| Teraspeed Modeling Services.
| http://www.teraspeedlabs.com
[IBIS Ver]   4.0
[Comment Char] |_char
[File Name]   lpc54114j256bd64.ibs
[File Rev]   3.0
[Source]  Measured and created by Teraspeed Labs
[Date]   10-25-2017
[Notes]   Quality Check of this IBIS model: Model Passes IBIS Check
   Model parses into ICX IS. Simulation done with Hyperlynx.
   1. MIN TYP MAX information is based on Temperature and Voltage
   characteristics only.
   2. Package data measured using Tektronix IConnect Software.
[Disclaimer]
| Use: Teraspeed Labs ("Teraspeed") has
| licensed IBIS models to specific integrated circuit
| suppliers ("IC Vendors") for use and distribution as
| follows: Each IC Vendor may use IBIS Models, and distribute
| them to IC Vendor's customers to use solely for developing
| printed circuit board designs. Users of this model may
| modify the IBIS model to suit its specific applications but
| rights to derivative works and such modifications shall belong
| to Teraspeed. No other distribution of these materials is
| permitted.
| DISCLAIMER OF WARRANTY: UNLESS OTHERWISE AGREED TO IN WRITING
| TERASPEED DISCLAIMS AND USER WAIVES ALL WARRANTIES, EXPRESS
| OR IMPLIED, INCLUDING WARRANTIES OF MERCHANTABILITY AND
| FITNESS FOR A PARTICULAR PURPOSE. IN NO EVENT SHALL
| TERASPEED BE LIABLE FOR ANY DIRECT OR INDIRECT DAMAGES,
| WHETHER IN CONTRACT OR TORT, INCLUDING, WITHOUT LIMITATION,
| LOST PROFITS, BUSINESS INTERRUPTION, OR LOST INFORMATION
| ARISING OUT OF THE USE OF OR THE INABILITY TO USE THE MODEL,
| EVEN IF TERASPEED HAS BEEN ADVISED OF THE POSSIBILITY OF SUCH
| DAMAGES.
[Copyright]
| This file is the legal property of Teraspeed Labs Copyright(c) 2017.
| All other rights are reserved.
[Component] LPC54114J256BD64
[Manufacturer] NXP Semiconductors
| Data Sheet: Rev 1.2, 24 February 2016
[Package]
| variable   typ   min   max
| LQFP64/SOT314-2
R_pkg  6.050E-02  5.800E-02  6.500E-02
L_pkg  5.046E-09  4.850E-09  5.380E-09
C_pkg  2.675E-13  2.400E-13  3.000E-13
[Pin] signal_name  model_name  R_pin  L_pin C_pin
1   PIO0_23   pio0_23   6.500E-02   5.380E-09   3.000E-13
2   PIO0_24   pio0_24   6.300E-02   5.250E-09   2.900E-13
3   PIO0_25   pio0_25   6.200E-02   5.130E-09   2.800E-13
4   PIO0_26   pio0_26   6.000E-02   5.040E-09   2.700E-13
5   USB_DP   analog_io   5.900E-02   4.950E-09   2.600E-13
6   USB_DM   analog_io   5.900E-02   4.900E-09   2.500E-13
7   PIO1_16   pio1_16   5.800E-02   4.870E-09   2.500E-13
8   VDD   POWER   5.800E-02   4.850E-09   2.400E-13
9   VSS   GND   5.800E-02   4.850E-09   2.400E-13
10   PIO1_17   pio1_17   5.800E-02   4.870E-09   2.500E-13
11   PIO0_29/ADC0_0   pio0_29   5.900E-02   4.900E-09   2.500E-13
12   PIO0_30/ADC0_1   pio0_30   5.900E-02   4.950E-09   2.600E-13
13   PIO0_31/ADC0_2   pio0_31   6.000E-02   5.040E-09   2.700E-13
14   PIO1_0/ADC0_3   pio1_0   6.200E-02   5.130E-09   2.800E-13
15   PIO1_1/ADC0_4   pio1_1   6.300E-02   5.250E-09   2.900E-13
16   PIO1_2/ADC0_5   pio1_2   6.500E-02   5.380E-09   3.000E-13
17   PIO1_3/ADC0_6   pio1_3   6.500E-02   5.380E-09   3.000E-13
18   PIO1_4/ADC0_7   pio1_4   6.300E-02   5.250E-09   2.900E-13
19   PIO1_5/ADC0_8   pio1_5   6.200E-02   5.130E-09   2.800E-13
20   VSSA   GND   6.000E-02   5.040E-09   2.700E-13
21   VREFN   GND   5.900E-02   4.950E-09   2.600E-13
22   VREFP   POWER   5.900E-02   4.900E-09   2.500E-13
23   VDDA   POWER   5.800E-02   4.870E-09   2.500E-13
24   VDD   POWER   5.800E-02   4.850E-09   2.400E-13
25   VSS   GND   5.800E-02   4.850E-09   2.400E-13
26   PIO1_6/ADC0_9   pio1_6   5.800E-02   4.870E-09   2.500E-13
27   PIO1_7/ADC0_10   pio1_7   5.900E-02   4.900E-09   2.500E-13
28   PIO1_8/ADC0_11   pio1_8   5.900E-02   4.950E-09   2.600E-13
29   PIO1_9   pio1_9   6.000E-02   5.040E-09   2.700E-13
30   PIO1_10   pio1_10   6.200E-02   5.130E-09   2.800E-13
31   PIO0_0   pio0_0   6.300E-02   5.250E-09   2.900E-13
32   PIO0_1   pio0_1   6.500E-02   5.380E-09   3.000E-13
33   RTCXIN   rtcxin   6.500E-02   5.380E-09   3.000E-13
34   VDD   POWER   6.300E-02   5.250E-09   2.900E-13
35   RTCXOUT   rtcxout   6.200E-02   5.130E-09   2.800E-13
36   PIO0_2   pio0_2   6.000E-02   5.040E-09   2.700E-13
37   PIO0_3   pio0_3   5.900E-02   4.950E-09   2.600E-13
38   PIO0_4   pio0_4   5.900E-02   4.900E-09   2.500E-13
39   PIO0_5   pio0_5   5.800E-02   4.870E-09   2.500E-13
40   PIO0_6   pio0_6   5.800E-02   4.850E-09   2.400E-13
41   PIO0_7   pio0_7   5.800E-02   4.850E-09   2.400E-13
42   PIO1_11   pio1_11   5.800E-02   4.870E-09   2.500E-13
43   PIO0_8   pio0_8   5.900E-02   4.900E-09   2.500E-13
44   PIO0_9   pio0_9   5.900E-02   4.950E-09   2.600E-13
45   PIO0_10   pio0_10   6.000E-02   5.040E-09   2.700E-13
46   PIO0_11   pio0_11   6.200E-02   5.130E-09   2.800E-13
47   PIO0_12   pio0_12   6.300E-02   5.250E-09   2.900E-13
48   PIO0_13   pio0_13   6.500E-02   5.380E-09   3.000E-13
49   PIO0_14/TCK   pio0_14   6.500E-02   5.380E-09   3.000E-13
50   PIO0_15/TDO   pio0_15   6.300E-02   5.250E-09   2.900E-13
51   PIO1_12   pio1_12   6.200E-02   5.130E-09   2.800E-13
52   SWCLK/PIO0_16   pio0_16   6.000E-02   5.040E-09   2.700E-13
53   SWDIO/PIO0_17   pio0_17   5.900E-02   4.950E-09   2.600E-13
54   PIO1_13   pio1_13   5.900E-02   4.900E-09   2.500E-13
55   VSS   GND   5.800E-02   4.870E-09   2.500E-13
56   VDD   POWER   5.800E-02   4.850E-09   2.400E-13
57   PIO1_14   pio1_14   5.800E-02   4.850E-09   2.400E-13
58   PIO0_18/*TRST   pio0_18   5.800E-02   4.870E-09   2.500E-13
59   PIO0_19/TDI   pio0_19   5.900E-02   4.900E-09   2.500E-13
60   PIO0_20/TMS   pio0_20   5.900E-02   4.950E-09   2.600E-13
61   PIO0_21   pio0_21   6.000E-02   5.040E-09   2.700E-13
62   PIO1_15   pio1_15   6.200E-02   5.130E-09   2.800E-13
63   PIO0_22   pio0_22   6.300E-02   5.250E-09   2.900E-13
64   *RESET   reset   6.500E-02   5.380E-09   3.000E-13
|**Open drain io pins
[Model Selector]   pio0_23
i2c_norm_hi_1.8v   i2c norm mode,hi drv,Open Drain io,1.8V
i2c_norm_hi_2.5v   i2c norm mode,hi drv,Open Drain io,2.5V
i2c_norm_hi_3.3v   i2c norm mode,hi drv,Open Drain io,3.3V
i2c_norm_lo_1.8v   i2c norm mode,lo drv,Open Drain io,1.8V
i2c_norm_lo_2.5v   i2c norm mode,lo drv,Open Drain io,2.5V
i2c_norm_lo_3.3v   i2c norm mode,lo drv,Open Drain io,3.3V
[Model Selector]   pio0_24
i2c_norm_hi_1.8v   i2c norm mode,hi drv,Open Drain io,1.8V
i2c_norm_hi_2.5v   i2c norm mode,hi drv,Open Drain io,2.5V
i2c_norm_hi_3.3v   i2c norm mode,hi drv,Open Drain io,3.3V
i2c_norm_lo_1.8v   i2c norm mode,lo drv,Open Drain io,1.8V
i2c_norm_lo_2.5v   i2c norm mode,lo drv,Open Drain io,2.5V
i2c_norm_lo_3.3v   i2c norm mode,lo drv,Open Drain io,3.3V
[Model Selector]   pio0_25
i2c_norm_hi_1.8v   i2c norm mode,hi drv,Open Drain io,1.8V
i2c_norm_hi_2.5v   i2c norm mode,hi drv,Open Drain io,2.5V
i2c_norm_hi_3.3v   i2c norm mode,hi drv,Open Drain io,3.3V
i2c_norm_lo_1.8v   i2c norm mode,lo drv,Open Drain io,1.8V
i2c_norm_lo_2.5v   i2c norm mode,lo drv,Open Drain io,2.5V
i2c_norm_lo_3.3v   i2c norm mode,lo drv,Open Drain io,3.3V
[Model Selector]   pio0_26
i2c_norm_hi_1.8v   i2c norm mode,hi drv,Open Drain io,1.8V
i2c_norm_hi_2.5v   i2c norm mode,hi drv,Open Drain io,2.5V
i2c_norm_hi_3.3v   i2c norm mode,hi drv,Open Drain io,3.3V
i2c_norm_lo_1.8v   i2c norm mode,lo drv,Open Drain io,1.8V
i2c_norm_lo_2.5v   i2c norm mode,lo drv,Open Drain io,2.5V
i2c_norm_lo_3.3v   i2c norm mode,lo drv,Open Drain io,3.3V
|**Standard io pins,5Vtol
[Model Selector]   pio0_0
pio_1.8v   GP io,1.8V
pio_2.5v   GP io,2.5V
pio_3.3v   GP io,3.3V
pio_1.8v_pd   GP io,pd,1.8V
pio_2.5v_pd   GP io,pd,2.5V
pio_3.3v_pd   GP io,pd,3.3V
pio_1.8v_pu   GP io,pu,1.8V | Pwrup Default
pio_2.5v_pu   GP io,pu,2.5V | Pwrup Default
pio_3.3v_pu   GP io,pu,3.3V | Pwrup Default
pio_fast_1.8v   GP io,fast slew,1.8V
pio_fast_2.5v   GP io,fast slew,2.5V
pio_fast_3.3v   GP io,fast slew,3.3V
pio_fast_1.8v_pd   GP io,fast slew,pd,1.8V
pio_fast_2.5v_pd   GP io,fast slew,pd,2.5V
pio_fast_3.3v_pd   GP io,fast slew,pd,3.3V
pio_fast_1.8v_pu   GP io,fast slew,pu,1.8V
pio_fast_2.5v_pu   GP io,fast slew,pu,2.5V
pio_fast_3.3v_pu   GP io,fast slew,pu,3.3V
[Model Selector]   pio0_1
pio_1.8v   GP io,1.8V
pio_2.5v   GP io,2.5V
pio_3.3v   GP io,3.3V
pio_1.8v_pd   GP io,pd,1.8V
pio_2.5v_pd   GP io,pd,2.5V
pio_3.3v_pd   GP io,pd,3.3V
pio_1.8v_pu   GP io,pu,1.8V | Pwrup Default
pio_2.5v_pu   GP io,pu,2.5V | Pwrup Default
pio_3.3v_pu   GP io,pu,3.3V | Pwrup Default
pio_fast_1.8v   GP io,fast slew,1.8V
pio_fast_2.5v   GP io,fast slew,2.5V
pio_fast_3.3v   GP io,fast slew,3.3V
pio_fast_1.8v_pd   GP io,fast slew,pd,1.8V
pio_fast_2.5v_pd   GP io,fast slew,pd,2.5V
pio_fast_3.3v_pd   GP io,fast slew,pd,3.3V
pio_fast_1.8v_pu   GP io,fast slew,pu,1.8V
pio_fast_2.5v_pu   GP io,fast slew,pu,2.5V
pio_fast_3.3v_pu   GP io,fast slew,pu,3.3V
[Model Selector]   pio0_2
pio_1.8v   GP io,1.8V
pio_2.5v   GP io,2.5V
pio_3.3v   GP io,3.3V
pio_1.8v_pd   GP io,pd,1.8V
pio_2.5v_pd   GP io,pd,2.5V
pio_3.3v_pd   GP io,pd,3.3V
pio_1.8v_pu   GP io,pu,1.8V | Pwrup Default
pio_2.5v_pu   GP io,pu,2.5V | Pwrup Default
pio_3.3v_pu   GP io,pu,3.3V | Pwrup Default
pio_fast_1.8v   GP io,fast slew,1.8V
pio_fast_2.5v   GP io,fast slew,2.5V
pio_fast_3.3v   GP io,fast slew,3.3V
pio_fast_1.8v_pd   GP io,fast slew,pd,1.8V
pio_fast_2.5v_pd   GP io,fast slew,pd,2.5V
pio_fast_3.3v_pd   GP io,fast slew,pd,3.3V
pio_fast_1.8v_pu   GP io,fast slew,pu,1.8V
pio_fast_2.5v_pu   GP io,fast slew,pu,2.5V
pio_fast_3.3v_pu   GP io,fast slew,pu,3.3V
[Model Selector]   pio0_3
pio_1.8v   GP io,1.8V
pio_2.5v   GP io,2.5V
pio_3.3v   GP io,3.3V
pio_1.8v_pd   GP io,pd,1.8V
pio_2.5v_pd   GP io,pd,2.5V
pio_3.3v_pd   GP io,pd,3.3V
pio_1.8v_pu   GP io,pu,1.8V | Pwrup Default
pio_2.5v_pu   GP io,pu,2.5V | Pwrup Default
pio_3.3v_pu   GP io,pu,3.3V | Pwrup Default
pio_fast_1.8v   GP io,fast slew,1.8V
pio_fast_2.5v   GP io,fast slew,2.5V
pio_fast_3.3v   GP io,fast slew,3.3V
pio_fast_1.8v_pd   GP io,fast slew,pd,1.8V
pio_fast_2.5v_pd   GP io,fast slew,pd,2.5V
pio_fast_3.3v_pd   GP io,fast slew,pd,3.3V
pio_fast_1.8v_pu   GP io,fast slew,pu,1.8V
pio_fast_2.5v_pu   GP io,fast slew,pu,2.5V
pio_fast_3.3v_pu   GP io,fast slew,pu,3.3V
[Model Selector]   pio0_4
pio_1.8v   GP io 1.8V | Pwrup Default
pio_2.5v   GP io 2.5V | Pwrup Default
pio_3.3v   GP io 3.3V | Pwrup Default
pio_1.8v_pu   GP io 1.8V with pullup
pio_2.5v_pu   GP io 2.5V with pullup
pio_3.3v_pu   GP io 3.3V with pullup
[Model Selector]   pio0_5
pio_1.8v   GP io,1.8V
pio_2.5v   GP io,2.5V
pio_3.3v   GP io,3.3V
pio_1.8v_pd   GP io,pd,1.8V
pio_2.5v_pd   GP io,pd,2.5V
pio_3.3v_pd   GP io,pd,3.3V
pio_1.8v_pu   GP io,pu,1.8V | Pwrup Default
pio_2.5v_pu   GP io,pu,2.5V | Pwrup Default
pio_3.3v_pu   GP io,pu,3.3V | Pwrup Default
pio_fast_1.8v   GP io,fast slew,1.8V
pio_fast_2.5v   GP io,fast slew,2.5V
pio_fast_3.3v   GP io,fast slew,3.3V
pio_fast_1.8v_pd   GP io,fast slew,pd,1.8V
pio_fast_2.5v_pd   GP io,fast slew,pd,2.5V
pio_fast_3.3v_pd   GP io,fast slew,pd,3.3V
pio_fast_1.8v_pu   GP io,fast slew,pu,1.8V
pio_fast_2.5v_pu   GP io,fast slew,pu,2.5V
pio_fast_3.3v_pu   GP io,fast slew,pu,3.3V
[Model Selector]   pio0_6
pio_1.8v   GP io,1.8V
pio_2.5v   GP io,2.5V
pio_3.3v   GP io,3.3V
pio_1.8v_pd   GP io,pd,1.8V
pio_2.5v_pd   GP io,pd,2.5V
pio_3.3v_pd   GP io,pd,3.3V
pio_1.8v_pu   GP io,pu,1.8V | Pwrup Default
pio_2.5v_pu   GP io,pu,2.5V | Pwrup Default
pio_3.3v_pu   GP io,pu,3.3V | Pwrup Default
pio_fast_1.8v   GP io,fast slew,1.8V
pio_fast_2.5v   GP io,fast slew,2.5V
pio_fast_3.3v   GP io,fast slew,3.3V
pio_fast_1.8v_pd   GP io,fast slew,pd,1.8V
pio_fast_2.5v_pd   GP io,fast slew,pd,2.5V
pio_fast_3.3v_pd   GP io,fast slew,pd,3.3V
pio_fast_1.8v_pu   GP io,fast slew,pu,1.8V
pio_fast_2.5v_pu   GP io,fast slew,pu,2.5V
pio_fast_3.3v_pu   GP io,fast slew,pu,3.3V
[Model Selector]   pio0_7
pio_1.8v   GP io,1.8V
pio_2.5v   GP io,2.5V
pio_3.3v   GP io,3.3V
pio_1.8v_pd   GP io,pd,1.8V
pio_2.5v_pd   GP io,pd,2.5V
pio_3.3v_pd   GP io,pd,3.3V
pio_1.8v_pu   GP io,pu,1.8V | Pwrup Default
pio_2.5v_pu   GP io,pu,2.5V | Pwrup Default
pio_3.3v_pu   GP io,pu,3.3V | Pwrup Default
pio_fast_1.8v   GP io,fast slew,1.8V
pio_fast_2.5v   GP io,fast slew,2.5V
pio_fast_3.3v   GP io,fast slew,3.3V
pio_fast_1.8v_pd   GP io,fast slew,pd,1.8V
pio_fast_2.5v_pd   GP io,fast slew,pd,2.5V
pio_fast_3.3v_pd   GP io,fast slew,pd,3.3V
pio_fast_1.8v_pu   GP io,fast slew,pu,1.8V
pio_fast_2.5v_pu   GP io,fast slew,pu,2.5V
pio_fast_3.3v_pu   GP io,fast slew,pu,3.3V
[Model Selector]   pio0_8
pio_1.8v   GP io 1.8V | Pwrup Default
pio_2.5v   GP io 2.5V | Pwrup Default
pio_3.3v   GP io 3.3V | Pwrup Default
pio_1.8v_pu   GP io 1.8V with pullup
pio_2.5v_pu   GP io 2.5V with pullup
pio_3.3v_pu   GP io 3.3V with pullup
[Model Selector]   pio0_9
pio_1.8v   GP io,1.8V
pio_2.5v   GP io,2.5V
pio_3.3v   GP io,3.3V
pio_1.8v_pd   GP io,pd,1.8V
pio_2.5v_pd   GP io,pd,2.5V
pio_3.3v_pd   GP io,pd,3.3V
pio_1.8v_pu   GP io,pu,1.8V | Pwrup Default
pio_2.5v_pu   GP io,pu,2.5V | Pwrup Default
pio_3.3v_pu   GP io,pu,3.3V | Pwrup Default
pio_fast_1.8v   GP io,fast slew,1.8V
pio_fast_2.5v   GP io,fast slew,2.5V
pio_fast_3.3v   GP io,fast slew,3.3V
pio_fast_1.8v_pd   GP io,fast slew,pd,1.8V
pio_fast_2.5v_pd   GP io,fast slew,pd,2.5V
pio_fast_3.3v_pd   GP io,fast slew,pd,3.3V
pio_fast_1.8v_pu   GP io,fast slew,pu,1.8V
pio_fast_2.5v_pu   GP io,fast slew,pu,2.5V
pio_fast_3.3v_pu   GP io,fast slew,pu,3.3V
[Model Selector]   pio0_10
pio_1.8v   GP io,1.8V
pio_2.5v   GP io,2.5V
pio_3.3v   GP io,3.3V
pio_1.8v_pd   GP io,pd,1.8V
pio_2.5v_pd   GP io,pd,2.5V
pio_3.3v_pd   GP io,pd,3.3V
pio_1.8v_pu   GP io,pu,1.8V | Pwrup Default
pio_2.5v_pu   GP io,pu,2.5V | Pwrup Default
pio_3.3v_pu   GP io,pu,3.3V | Pwrup Default
pio_fast_1.8v   GP io,fast slew,1.8V
pio_fast_2.5v   GP io,fast slew,2.5V
pio_fast_3.3v   GP io,fast slew,3.3V
pio_fast_1.8v_pd   GP io,fast slew,pd,1.8V
pio_fast_2.5v_pd   GP io,fast slew,pd,2.5V
pio_fast_3.3v_pd   GP io,fast slew,pd,3.3V
pio_fast_1.8v_pu   GP io,fast slew,pu,1.8V
pio_fast_2.5v_pu   GP io,fast slew,pu,2.5V
pio_fast_3.3v_pu   GP io,fast slew,pu,3.3V
[Model Selector]   pio0_11
pio_1.8v   GP io,1.8V
pio_2.5v   GP io,2.5V
pio_3.3v   GP io,3.3V
pio_1.8v_pd   GP io,pd,1.8V
pio_2.5v_pd   GP io,pd,2.5V
pio_3.3v_pd   GP io,pd,3.3V
pio_1.8v_pu   GP io,pu,1.8V | Pwrup Default
pio_2.5v_pu   GP io,pu,2.5V | Pwrup Default
pio_3.3v_pu   GP io,pu,3.3V | Pwrup Default
pio_fast_1.8v   GP io,fast slew,1.8V
pio_fast_2.5v   GP io,fast slew,2.5V
pio_fast_3.3v   GP io,fast slew,3.3V
pio_fast_1.8v_pd   GP io,fast slew,pd,1.8V
pio_fast_2.5v_pd   GP io,fast slew,pd,2.5V
pio_fast_3.3v_pd   GP io,fast slew,pd,3.3V
pio_fast_1.8v_pu   GP io,fast slew,pu,1.8V
pio_fast_2.5v_pu   GP io,fast slew,pu,2.5V
pio_fast_3.3v_pu   GP io,fast slew,pu,3.3V
[Model Selector]   pio0_12
pio_1.8v   GP io,1.8V
pio_2.5v   GP io,2.5V
pio_3.3v   GP io,3.3V
pio_1.8v_pd   GP io,pd,1.8V
pio_2.5v_pd   GP io,pd,2.5V
pio_3.3v_pd   GP io,pd,3.3V
pio_1.8v_pu   GP io,pu,1.8V | Pwrup Default
pio_2.5v_pu   GP io,pu,2.5V | Pwrup Default
pio_3.3v_pu   GP io,pu,3.3V | Pwrup Default
pio_fast_1.8v   GP io,fast slew,1.8V
pio_fast_2.5v   GP io,fast slew,2.5V
pio_fast_3.3v   GP io,fast slew,3.3V
pio_fast_1.8v_pd   GP io,fast slew,pd,1.8V
pio_fast_2.5v_pd   GP io,fast slew,pd,2.5V
pio_fast_3.3v_pd   GP io,fast slew,pd,3.3V
pio_fast_1.8v_pu   GP io,fast slew,pu,1.8V
pio_fast_2.5v_pu   GP io,fast slew,pu,2.5V
pio_fast_3.3v_pu   GP io,fast slew,pu,3.3V
[Model Selector]   pio0_13
pio_1.8v   GP io,1.8V
pio_2.5v   GP io,2.5V
pio_3.3v   GP io,3.3V
pio_1.8v_pd   GP io,pd,1.8V
pio_2.5v_pd   GP io,pd,2.5V
pio_3.3v_pd   GP io,pd,3.3V
pio_1.8v_pu   GP io,pu,1.8V | Pwrup Default
pio_2.5v_pu   GP io,pu,2.5V | Pwrup Default
pio_3.3v_pu   GP io,pu,3.3V | Pwrup Default
pio_fast_1.8v   GP io,fast slew,1.8V
pio_fast_2.5v   GP io,fast slew,2.5V
pio_fast_3.3v   GP io,fast slew,3.3V
pio_fast_1.8v_pd   GP io,fast slew,pd,1.8V
pio_fast_2.5v_pd   GP io,fast slew,pd,2.5V
pio_fast_3.3v_pd   GP io,fast slew,pd,3.3V
pio_fast_1.8v_pu   GP io,fast slew,pu,1.8V
pio_fast_2.5v_pu   GP io,fast slew,pu,2.5V
pio_fast_3.3v_pu   GP io,fast slew,pu,3.3V
[Model Selector]   pio0_14
pio_1.8v   GP io,1.8V
pio_2.5v   GP io,2.5V
pio_3.3v   GP io,3.3V
pio_1.8v_pd   GP io,pd,1.8V
pio_2.5v_pd   GP io,pd,2.5V
pio_3.3v_pd   GP io,pd,3.3V
pio_1.8v_pu   GP io,pu,1.8V | Pwrup Default
pio_2.5v_pu   GP io,pu,2.5V | Pwrup Default
pio_3.3v_pu   GP io,pu,3.3V | Pwrup Default
pio_fast_1.8v   GP io,fast slew,1.8V
pio_fast_2.5v   GP io,fast slew,2.5V
pio_fast_3.3v   GP io,fast slew,3.3V
pio_fast_1.8v_pd   GP io,fast slew,pd,1.8V
pio_fast_2.5v_pd   GP io,fast slew,pd,2.5V
pio_fast_3.3v_pd   GP io,fast slew,pd,3.3V
pio_fast_1.8v_pu   GP io,fast slew,pu,1.8V
pio_fast_2.5v_pu   GP io,fast slew,pu,2.5V
pio_fast_3.3v_pu   GP io,fast slew,pu,3.3V
[Model Selector]   pio0_15
pio_1.8v   GP io,1.8V
pio_2.5v   GP io,2.5V
pio_3.3v   GP io,3.3V
pio_1.8v_pd   GP io,pd,1.8V
pio_2.5v_pd   GP io,pd,2.5V
pio_3.3v_pd   GP io,pd,3.3V
pio_1.8v_pu   GP io,pu,1.8V | Pwrup Default
pio_2.5v_pu   GP io,pu,2.5V | Pwrup Default
pio_3.3v_pu   GP io,pu,3.3V | Pwrup Default
pio_fast_1.8v   GP io,fast slew,1.8V
pio_fast_2.5v   GP io,fast slew,2.5V
pio_fast_3.3v   GP io,fast slew,3.3V
pio_fast_1.8v_pd   GP io,fast slew,pd,1.8V
pio_fast_2.5v_pd   GP io,fast slew,pd,2.5V
pio_fast_3.3v_pd   GP io,fast slew,pd,3.3V
pio_fast_1.8v_pu   GP io,fast slew,pu,1.8V
pio_fast_2.5v_pu   GP io,fast slew,pu,2.5V
pio_fast_3.3v_pu   GP io,fast slew,pu,3.3V
[Model Selector]   pio0_16
pio_1.8v   GP io,1.8V
pio_2.5v   GP io,2.5V
pio_3.3v   GP io,3.3V
pio_1.8v_pd   GP io,pd,1.8V
pio_2.5v_pd   GP io,pd,2.5V
pio_3.3v_pd   GP io,pd,3.3V
pio_1.8v_pu   GP io,pu,1.8V | Pwrup Default
pio_2.5v_pu   GP io,pu,2.5V | Pwrup Default
pio_3.3v_pu   GP io,pu,3.3V | Pwrup Default
pio_fast_1.8v   GP io,fast slew,1.8V
pio_fast_2.5v   GP io,fast slew,2.5V
pio_fast_3.3v   GP io,fast slew,3.3V
pio_fast_1.8v_pd   GP io,fast slew,pd,1.8V
pio_fast_2.5v_pd   GP io,fast slew,pd,2.5V
pio_fast_3.3v_pd   GP io,fast slew,pd,3.3V
pio_fast_1.8v_pu   GP io,fast slew,pu,1.8V
pio_fast_2.5v_pu   GP io,fast slew,pu,2.5V
pio_fast_3.3v_pu   GP io,fast slew,pu,3.3V
[Model Selector]   pio0_17
pio_1.8v   GP io,1.8V
pio_2.5v   GP io,2.5V
pio_3.3v   GP io,3.3V
pio_1.8v_pd   GP io,pd,1.8V
pio_2.5v_pd   GP io,pd,2.5V
pio_3.3v_pd   GP io,pd,3.3V
pio_1.8v_pu   GP io,pu,1.8V | Pwrup Default
pio_2.5v_pu   GP io,pu,2.5V | Pwrup Default
pio_3.3v_pu   GP io,pu,3.3V | Pwrup Default
pio_fast_1.8v   GP io,fast slew,1.8V
pio_fast_2.5v   GP io,fast slew,2.5V
pio_fast_3.3v   GP io,fast slew,3.3V
pio_fast_1.8v_pd   GP io,fast slew,pd,1.8V
pio_fast_2.5v_pd   GP io,fast slew,pd,2.5V
pio_fast_3.3v_pd   GP io,fast slew,pd,3.3V
pio_fast_1.8v_pu   GP io,fast slew,pu,1.8V
pio_fast_2.5v_pu   GP io,fast slew,pu,2.5V
pio_fast_3.3v_pu   GP io,fast slew,pu,3.3V
[Model Selector]   pio0_18
pio_1.8v   GP io,1.8V
pio_2.5v   GP io,2.5V
pio_3.3v   GP io,3.3V
pio_1.8v_pd   GP io,pd,1.8V
pio_2.5v_pd   GP io,pd,2.5V
pio_3.3v_pd   GP io,pd,3.3V
pio_1.8v_pu   GP io,pu,1.8V | Pwrup Default
pio_2.5v_pu   GP io,pu,2.5V | Pwrup Default
pio_3.3v_pu   GP io,pu,3.3V | Pwrup Default
pio_fast_1.8v   GP io,fast slew,1.8V
pio_fast_2.5v   GP io,fast slew,2.5V
pio_fast_3.3v   GP io,fast slew,3.3V
pio_fast_1.8v_pd   GP io,fast slew,pd,1.8V
pio_fast_2.5v_pd   GP io,fast slew,pd,2.5V
pio_fast_3.3v_pd   GP io,fast slew,pd,3.3V
pio_fast_1.8v_pu   GP io,fast slew,pu,1.8V
pio_fast_2.5v_pu   GP io,fast slew,pu,2.5V
pio_fast_3.3v_pu   GP io,fast slew,pu,3.3V
[Model Selector]   pio0_19
pio_1.8v   GP io,1.8V
pio_2.5v   GP io,2.5V
pio_3.3v   GP io,3.3V
pio_1.8v_pd   GP io,pd,1.8V
pio_2.5v_pd   GP io,pd,2.5V
pio_3.3v_pd   GP io,pd,3.3V
pio_1.8v_pu   GP io,pu,1.8V | Pwrup Default
pio_2.5v_pu   GP io,pu,2.5V | Pwrup Default
pio_3.3v_pu   GP io,pu,3.3V | Pwrup Default
pio_fast_1.8v   GP io,fast slew,1.8V
pio_fast_2.5v   GP io,fast slew,2.5V
pio_fast_3.3v   GP io,fast slew,3.3V
pio_fast_1.8v_pd   GP io,fast slew,pd,1.8V
pio_fast_2.5v_pd   GP io,fast slew,pd,2.5V
pio_fast_3.3v_pd   GP io,fast slew,pd,3.3V
pio_fast_1.8v_pu   GP io,fast slew,pu,1.8V
pio_fast_2.5v_pu   GP io,fast slew,pu,2.5V
pio_fast_3.3v_pu   GP io,fast slew,pu,3.3V
[Model Selector]   pio0_20
pio_1.8v   GP io,1.8V
pio_2.5v   GP io,2.5V
pio_3.3v   GP io,3.3V
pio_1.8v_pd   GP io,pd,1.8V
pio_2.5v_pd   GP io,pd,2.5V
pio_3.3v_pd   GP io,pd,3.3V
pio_1.8v_pu   GP io,pu,1.8V | Pwrup Default
pio_2.5v_pu   GP io,pu,2.5V | Pwrup Default
pio_3.3v_pu   GP io,pu,3.3V | Pwrup Default
pio_fast_1.8v   GP io,fast slew,1.8V
pio_fast_2.5v   GP io,fast slew,2.5V
pio_fast_3.3v   GP io,fast slew,3.3V
pio_fast_1.8v_pd   GP io,fast slew,pd,1.8V
pio_fast_2.5v_pd   GP io,fast slew,pd,2.5V
pio_fast_3.3v_pd   GP io,fast slew,pd,3.3V
pio_fast_1.8v_pu   GP io,fast slew,pu,1.8V
pio_fast_2.5v_pu   GP io,fast slew,pu,2.5V
pio_fast_3.3v_pu   GP io,fast slew,pu,3.3V
[Model Selector]   pio0_21
pio_1.8v   GP io,1.8V
pio_2.5v   GP io,2.5V
pio_3.3v   GP io,3.3V
pio_1.8v_pd   GP io,pd,1.8V
pio_2.5v_pd   GP io,pd,2.5V
pio_3.3v_pd   GP io,pd,3.3V
pio_1.8v_pu   GP io,pu,1.8V | Pwrup Default
pio_2.5v_pu   GP io,pu,2.5V | Pwrup Default
pio_3.3v_pu   GP io,pu,3.3V | Pwrup Default
pio_fast_1.8v   GP io,fast slew,1.8V
pio_fast_2.5v   GP io,fast slew,2.5V
pio_fast_3.3v   GP io,fast slew,3.3V
pio_fast_1.8v_pd   GP io,fast slew,pd,1.8V
pio_fast_2.5v_pd   GP io,fast slew,pd,2.5V
pio_fast_3.3v_pd   GP io,fast slew,pd,3.3V
pio_fast_1.8v_pu   GP io,fast slew,pu,1.8V
pio_fast_2.5v_pu   GP io,fast slew,pu,2.5V
pio_fast_3.3v_pu   GP io,fast slew,pu,3.3V
[Model Selector]   pio0_22
pio_1.8v   GP io,1.8V
pio_2.5v   GP io,2.5V
pio_3.3v   GP io,3.3V
pio_1.8v_pd   GP io,pd,1.8V
pio_2.5v_pd   GP io,pd,2.5V
pio_3.3v_pd   GP io,pd,3.3V
pio_1.8v_pu   GP io,pu,1.8V | Pwrup Default
pio_2.5v_pu   GP io,pu,2.5V | Pwrup Default
pio_3.3v_pu   GP io,pu,3.3V | Pwrup Default
pio_fast_1.8v   GP io,fast slew,1.8V
pio_fast_2.5v   GP io,fast slew,2.5V
pio_fast_3.3v   GP io,fast slew,3.3V
pio_fast_1.8v_pd   GP io,fast slew,pd,1.8V
pio_fast_2.5v_pd   GP io,fast slew,pd,2.5V
pio_fast_3.3v_pd   GP io,fast slew,pd,3.3V
pio_fast_1.8v_pu   GP io,fast slew,pu,1.8V
pio_fast_2.5v_pu   GP io,fast slew,pu,2.5V
pio_fast_3.3v_pu   GP io,fast slew,pu,3.3V
[Model Selector]   pio1_9
pio_1.8v   GP io,1.8V
pio_2.5v   GP io,2.5V
pio_3.3v   GP io,3.3V
pio_1.8v_pd   GP io,pd,1.8V
pio_2.5v_pd   GP io,pd,2.5V
pio_3.3v_pd   GP io,pd,3.3V
pio_1.8v_pu   GP io,pu,1.8V | Pwrup Default
pio_2.5v_pu   GP io,pu,2.5V | Pwrup Default
pio_3.3v_pu   GP io,pu,3.3V | Pwrup Default
pio_fast_1.8v   GP io,fast slew,1.8V
pio_fast_2.5v   GP io,fast slew,2.5V
pio_fast_3.3v   GP io,fast slew,3.3V
pio_fast_1.8v_pd   GP io,fast slew,pd,1.8V
pio_fast_2.5v_pd   GP io,fast slew,pd,2.5V
pio_fast_3.3v_pd   GP io,fast slew,pd,3.3V
pio_fast_1.8v_pu   GP io,fast slew,pu,1.8V
pio_fast_2.5v_pu   GP io,fast slew,pu,2.5V
pio_fast_3.3v_pu   GP io,fast slew,pu,3.3V
[Model Selector]   pio1_10
pio_1.8v   GP io,1.8V
pio_2.5v   GP io,2.5V
pio_3.3v   GP io,3.3V
pio_1.8v_pd   GP io,pd,1.8V
pio_2.5v_pd   GP io,pd,2.5V
pio_3.3v_pd   GP io,pd,3.3V
pio_1.8v_pu   GP io,pu,1.8V | Pwrup Default
pio_2.5v_pu   GP io,pu,2.5V | Pwrup Default
pio_3.3v_pu   GP io,pu,3.3V | Pwrup Default
pio_fast_1.8v   GP io,fast slew,1.8V
pio_fast_2.5v   GP io,fast slew,2.5V
pio_fast_3.3v   GP io,fast slew,3.3V
pio_fast_1.8v_pd   GP io,fast slew,pd,1.8V
pio_fast_2.5v_pd   GP io,fast slew,pd,2.5V
pio_fast_3.3v_pd   GP io,fast slew,pd,3.3V
pio_fast_1.8v_pu   GP io,fast slew,pu,1.8V
pio_fast_2.5v_pu   GP io,fast slew,pu,2.5V
pio_fast_3.3v_pu   GP io,fast slew,pu,3.3V
[Model Selector]   pio1_11
pio_1.8v   GP io,1.8V
pio_2.5v   GP io,2.5V
pio_3.3v   GP io,3.3V
pio_1.8v_pd   GP io,pd,1.8V
pio_2.5v_pd   GP io,pd,2.5V
pio_3.3v_pd   GP io,pd,3.3V
pio_1.8v_pu   GP io,pu,1.8V | Pwrup Default
pio_2.5v_pu   GP io,pu,2.5V | Pwrup Default
pio_3.3v_pu   GP io,pu,3.3V | Pwrup Default
pio_fast_1.8v   GP io,fast slew,1.8V
pio_fast_2.5v   GP io,fast slew,2.5V
pio_fast_3.3v   GP io,fast slew,3.3V
pio_fast_1.8v_pd   GP io,fast slew,pd,1.8V
pio_fast_2.5v_pd   GP io,fast slew,pd,2.5V
pio_fast_3.3v_pd   GP io,fast slew,pd,3.3V
pio_fast_1.8v_pu   GP io,fast slew,pu,1.8V
pio_fast_2.5v_pu   GP io,fast slew,pu,2.5V
pio_fast_3.3v_pu   GP io,fast slew,pu,3.3V
[Model Selector]   pio1_12
pio_1.8v   GP io,1.8V
pio_2.5v   GP io,2.5V
pio_3.3v   GP io,3.3V
pio_1.8v_pd   GP io,pd,1.8V
pio_2.5v_pd   GP io,pd,2.5V
pio_3.3v_pd   GP io,pd,3.3V
pio_1.8v_pu   GP io,pu,1.8V | Pwrup Default
pio_2.5v_pu   GP io,pu,2.5V | Pwrup Default
pio_3.3v_pu   GP io,pu,3.3V | Pwrup Default
pio_fast_1.8v   GP io,fast slew,1.8V
pio_fast_2.5v   GP io,fast slew,2.5V
pio_fast_3.3v   GP io,fast slew,3.3V
pio_fast_1.8v_pd   GP io,fast slew,pd,1.8V
pio_fast_2.5v_pd   GP io,fast slew,pd,2.5V
pio_fast_3.3v_pd   GP io,fast slew,pd,3.3V
pio_fast_1.8v_pu   GP io,fast slew,pu,1.8V
pio_fast_2.5v_pu   GP io,fast slew,pu,2.5V
pio_fast_3.3v_pu   GP io,fast slew,pu,3.3V
[Model Selector]   pio1_13
pio_1.8v   GP io,1.8V
pio_2.5v   GP io,2.5V
pio_3.3v   GP io,3.3V
pio_1.8v_pd   GP io,pd,1.8V
pio_2.5v_pd   GP io,pd,2.5V
pio_3.3v_pd   GP io,pd,3.3V
pio_1.8v_pu   GP io,pu,1.8V | Pwrup Default
pio_2.5v_pu   GP io,pu,2.5V | Pwrup Default
pio_3.3v_pu   GP io,pu,3.3V | Pwrup Default
pio_fast_1.8v   GP io,fast slew,1.8V
pio_fast_2.5v   GP io,fast slew,2.5V
pio_fast_3.3v   GP io,fast slew,3.3V
pio_fast_1.8v_pd   GP io,fast slew,pd,1.8V
pio_fast_2.5v_pd   GP io,fast slew,pd,2.5V
pio_fast_3.3v_pd   GP io,fast slew,pd,3.3V
pio_fast_1.8v_pu   GP io,fast slew,pu,1.8V
pio_fast_2.5v_pu   GP io,fast slew,pu,2.5V
pio_fast_3.3v_pu   GP io,fast slew,pu,3.3V
[Model Selector]   pio1_14
pio_1.8v   GP io,1.8V
pio_2.5v   GP io,2.5V
pio_3.3v   GP io,3.3V
pio_1.8v_pd   GP io,pd,1.8V
pio_2.5v_pd   GP io,pd,2.5V
pio_3.3v_pd   GP io,pd,3.3V
pio_1.8v_pu   GP io,pu,1.8V | Pwrup Default
pio_2.5v_pu   GP io,pu,2.5V | Pwrup Default
pio_3.3v_pu   GP io,pu,3.3V | Pwrup Default
pio_fast_1.8v   GP io,fast slew,1.8V
pio_fast_2.5v   GP io,fast slew,2.5V
pio_fast_3.3v   GP io,fast slew,3.3V
pio_fast_1.8v_pd   GP io,fast slew,pd,1.8V
pio_fast_2.5v_pd   GP io,fast slew,pd,2.5V
pio_fast_3.3v_pd   GP io,fast slew,pd,3.3V
pio_fast_1.8v_pu   GP io,fast slew,pu,1.8V
pio_fast_2.5v_pu   GP io,fast slew,pu,2.5V
pio_fast_3.3v_pu   GP io,fast slew,pu,3.3V
[Model Selector]   pio1_15
pio_1.8v   GP io,1.8V
pio_2.5v   GP io,2.5V
pio_3.3v   GP io,3.3V
pio_1.8v_pd   GP io,pd,1.8V
pio_2.5v_pd   GP io,pd,2.5V
pio_3.3v_pd   GP io,pd,3.3V
pio_1.8v_pu   GP io,pu,1.8V | Pwrup Default
pio_2.5v_pu   GP io,pu,2.5V | Pwrup Default
pio_3.3v_pu   GP io,pu,3.3V | Pwrup Default
pio_fast_1.8v   GP io,fast slew,1.8V
pio_fast_2.5v   GP io,fast slew,2.5V
pio_fast_3.3v   GP io,fast slew,3.3V
pio_fast_1.8v_pd   GP io,fast slew,pd,1.8V
pio_fast_2.5v_pd   GP io,fast slew,pd,2.5V
pio_fast_3.3v_pd   GP io,fast slew,pd,3.3V
pio_fast_1.8v_pu   GP io,fast slew,pu,1.8V
pio_fast_2.5v_pu   GP io,fast slew,pu,2.5V
pio_fast_3.3v_pu   GP io,fast slew,pu,3.3V
[Model Selector]   pio1_16
pio_1.8v   GP io,1.8V
pio_2.5v   GP io,2.5V
pio_3.3v   GP io,3.3V
pio_1.8v_pd   GP io,pd,1.8V
pio_2.5v_pd   GP io,pd,2.5V
pio_3.3v_pd   GP io,pd,3.3V
pio_1.8v_pu   GP io,pu,1.8V | Pwrup Default
pio_2.5v_pu   GP io,pu,2.5V | Pwrup Default
pio_3.3v_pu   GP io,pu,3.3V | Pwrup Default
pio_fast_1.8v   GP io,fast slew,1.8V
pio_fast_2.5v   GP io,fast slew,2.5V
pio_fast_3.3v   GP io,fast slew,3.3V
pio_fast_1.8v_pd   GP io,fast slew,pd,1.8V
pio_fast_2.5v_pd   GP io,fast slew,pd,2.5V
pio_fast_3.3v_pd   GP io,fast slew,pd,3.3V
pio_fast_1.8v_pu   GP io,fast slew,pu,1.8V
pio_fast_2.5v_pu   GP io,fast slew,pu,2.5V
pio_fast_3.3v_pu   GP io,fast slew,pu,3.3V
[Model Selector]   pio1_17
pio_1.8v   GP io,1.8V
pio_2.5v   GP io,2.5V
pio_3.3v   GP io,3.3V
pio_1.8v_pd   GP io,pd,1.8V
pio_2.5v_pd   GP io,pd,2.5V
pio_3.3v_pd   GP io,pd,3.3V
pio_1.8v_pu   GP io,pu,1.8V | Pwrup Default
pio_2.5v_pu   GP io,pu,2.5V | Pwrup Default
pio_3.3v_pu   GP io,pu,3.3V | Pwrup Default
pio_fast_1.8v   GP io,fast slew,1.8V
pio_fast_2.5v   GP io,fast slew,2.5V
pio_fast_3.3v   GP io,fast slew,3.3V
pio_fast_1.8v_pd   GP io,fast slew,pd,1.8V
pio_fast_2.5v_pd   GP io,fast slew,pd,2.5V
pio_fast_3.3v_pd   GP io,fast slew,pd,3.3V
pio_fast_1.8v_pu   GP io,fast slew,pu,1.8V
pio_fast_2.5v_pu   GP io,fast slew,pu,2.5V
pio_fast_3.3v_pu   GP io,fast slew,pu,3.3V
|**Standard io pins w/analog function
[Model Selector]   pio0_29
pio_1.8v   GP io,1.8V
pio_2.5v   GP io,2.5V
pio_3.3v   GP io,3.3V
pio_1.8v_pd   GP io,pd,1.8V
pio_2.5v_pd   GP io,pd,2.5V
pio_3.3v_pd   GP io,pd,3.3V
pio_1.8v_pu   GP io,pu,1.8V | Pwrup Default
pio_2.5v_pu   GP io,pu,2.5V | Pwrup Default
pio_3.3v_pu   GP io,pu,3.3V | Pwrup Default
pio_fast_1.8v   GP io,fast slew,1.8V
pio_fast_2.5v   GP io,fast slew,2.5V
pio_fast_3.3v   GP io,fast slew,3.3V
pio_fast_1.8v_pd   GP io,fast slew,pd,1.8V
pio_fast_2.5v_pd   GP io,fast slew,pd,2.5V
pio_fast_3.3v_pd   GP io,fast slew,pd,3.3V
pio_fast_1.8v_pu   GP io,fast slew,pu,1.8V
pio_fast_2.5v_pu   GP io,fast slew,pu,2.5V
pio_fast_3.3v_pu   GP io,fast slew,pu,3.3V
analog_1.8v   adc input 1.8v
analog_2.5v   adc input 2.5v
analog_3.3v   adc input 3.3v
[Model Selector]   pio0_30
pio_1.8v   GP io,1.8V
pio_2.5v   GP io,2.5V
pio_3.3v   GP io,3.3V
pio_1.8v_pd   GP io,pd,1.8V
pio_2.5v_pd   GP io,pd,2.5V
pio_3.3v_pd   GP io,pd,3.3V
pio_1.8v_pu   GP io,pu,1.8V | Pwrup Default
pio_2.5v_pu   GP io,pu,2.5V | Pwrup Default
pio_3.3v_pu   GP io,pu,3.3V | Pwrup Default
pio_fast_1.8v   GP io,fast slew,1.8V
pio_fast_2.5v   GP io,fast slew,2.5V
pio_fast_3.3v   GP io,fast slew,3.3V
pio_fast_1.8v_pd   GP io,fast slew,pd,1.8V
pio_fast_2.5v_pd   GP io,fast slew,pd,2.5V
pio_fast_3.3v_pd   GP io,fast slew,pd,3.3V
pio_fast_1.8v_pu   GP io,fast slew,pu,1.8V
pio_fast_2.5v_pu   GP io,fast slew,pu,2.5V
pio_fast_3.3v_pu   GP io,fast slew,pu,3.3V
analog_1.8v   adc input 1.8v
analog_2.5v   adc input 2.5v
analog_3.3v   adc input 3.3v
[Model Selector]   pio0_31
pio_1.8v   GP io,1.8V
pio_2.5v   GP io,2.5V
pio_3.3v   GP io,3.3V
pio_1.8v_pd   GP io,pd,1.8V
pio_2.5v_pd   GP io,pd,2.5V
pio_3.3v_pd   GP io,pd,3.3V
pio_1.8v_pu   GP io,pu,1.8V | Pwrup Default
pio_2.5v_pu   GP io,pu,2.5V | Pwrup Default
pio_3.3v_pu   GP io,pu,3.3V | Pwrup Default
pio_fast_1.8v   GP io,fast slew,1.8V
pio_fast_2.5v   GP io,fast slew,2.5V
pio_fast_3.3v   GP io,fast slew,3.3V
pio_fast_1.8v_pd   GP io,fast slew,pd,1.8V
pio_fast_2.5v_pd   GP io,fast slew,pd,2.5V
pio_fast_3.3v_pd   GP io,fast slew,pd,3.3V
pio_fast_1.8v_pu   GP io,fast slew,pu,1.8V
pio_fast_2.5v_pu   GP io,fast slew,pu,2.5V
pio_fast_3.3v_pu   GP io,fast slew,pu,3.3V
analog_1.8v   adc input 1.8v
analog_2.5v   adc input 2.5v
analog_3.3v   adc input 3.3v
[Model Selector]   pio1_0
pio_1.8v   GP io,1.8V
pio_2.5v   GP io,2.5V
pio_3.3v   GP io,3.3V
pio_1.8v_pd   GP io,pd,1.8V
pio_2.5v_pd   GP io,pd,2.5V
pio_3.3v_pd   GP io,pd,3.3V
pio_1.8v_pu   GP io,pu,1.8V | Pwrup Default
pio_2.5v_pu   GP io,pu,2.5V | Pwrup Default
pio_3.3v_pu   GP io,pu,3.3V | Pwrup Default
pio_fast_1.8v   GP io,fast slew,1.8V
pio_fast_2.5v   GP io,fast slew,2.5V
pio_fast_3.3v   GP io,fast slew,3.3V
pio_fast_1.8v_pd   GP io,fast slew,pd,1.8V
pio_fast_2.5v_pd   GP io,fast slew,pd,2.5V
pio_fast_3.3v_pd   GP io,fast slew,pd,3.3V
pio_fast_1.8v_pu   GP io,fast slew,pu,1.8V
pio_fast_2.5v_pu   GP io,fast slew,pu,2.5V
pio_fast_3.3v_pu   GP io,fast slew,pu,3.3V
analog_1.8v   adc input 1.8v
analog_2.5v   adc input 2.5v
analog_3.3v   adc input 3.3v
[Model Selector]   pio1_1
pio_1.8v   GP io,1.8V
pio_2.5v   GP io,2.5V
pio_3.3v   GP io,3.3V
pio_1.8v_pd   GP io,pd,1.8V
pio_2.5v_pd   GP io,pd,2.5V
pio_3.3v_pd   GP io,pd,3.3V
pio_1.8v_pu   GP io,pu,1.8V | Pwrup Default
pio_2.5v_pu   GP io,pu,2.5V | Pwrup Default
pio_3.3v_pu   GP io,pu,3.3V | Pwrup Default
pio_fast_1.8v   GP io,fast slew,1.8V
pio_fast_2.5v   GP io,fast slew,2.5V
pio_fast_3.3v   GP io,fast slew,3.3V
pio_fast_1.8v_pd   GP io,fast slew,pd,1.8V
pio_fast_2.5v_pd   GP io,fast slew,pd,2.5V
pio_fast_3.3v_pd   GP io,fast slew,pd,3.3V
pio_fast_1.8v_pu   GP io,fast slew,pu,1.8V
pio_fast_2.5v_pu   GP io,fast slew,pu,2.5V
pio_fast_3.3v_pu   GP io,fast slew,pu,3.3V
analog_1.8v   adc input 1.8v
analog_2.5v   adc input 2.5v
analog_3.3v   adc input 3.3v
[Model Selector]   pio1_2
pio_1.8v   GP io,1.8V
pio_2.5v   GP io,2.5V
pio_3.3v   GP io,3.3V
pio_1.8v_pd   GP io,pd,1.8V
pio_2.5v_pd   GP io,pd,2.5V
pio_3.3v_pd   GP io,pd,3.3V
pio_1.8v_pu   GP io,pu,1.8V | Pwrup Default
pio_2.5v_pu   GP io,pu,2.5V | Pwrup Default
pio_3.3v_pu   GP io,pu,3.3V | Pwrup Default
pio_fast_1.8v   GP io,fast slew,1.8V
pio_fast_2.5v   GP io,fast slew,2.5V
pio_fast_3.3v   GP io,fast slew,3.3V
pio_fast_1.8v_pd   GP io,fast slew,pd,1.8V
pio_fast_2.5v_pd   GP io,fast slew,pd,2.5V
pio_fast_3.3v_pd   GP io,fast slew,pd,3.3V
pio_fast_1.8v_pu   GP io,fast slew,pu,1.8V
pio_fast_2.5v_pu   GP io,fast slew,pu,2.5V
pio_fast_3.3v_pu   GP io,fast slew,pu,3.3V
analog_1.8v   adc input 1.8v
analog_2.5v   adc input 2.5v
analog_3.3v   adc input 3.3v
[Model Selector]   pio1_3
pio_1.8v   GP io,1.8V
pio_2.5v   GP io,2.5V
pio_3.3v   GP io,3.3V
pio_1.8v_pd   GP io,pd,1.8V
pio_2.5v_pd   GP io,pd,2.5V
pio_3.3v_pd   GP io,pd,3.3V
pio_1.8v_pu   GP io,pu,1.8V | Pwrup Default
pio_2.5v_pu   GP io,pu,2.5V | Pwrup Default
pio_3.3v_pu   GP io,pu,3.3V | Pwrup Default
pio_fast_1.8v   GP io,fast slew,1.8V
pio_fast_2.5v   GP io,fast slew,2.5V
pio_fast_3.3v   GP io,fast slew,3.3V
pio_fast_1.8v_pd   GP io,fast slew,pd,1.8V
pio_fast_2.5v_pd   GP io,fast slew,pd,2.5V
pio_fast_3.3v_pd   GP io,fast slew,pd,3.3V
pio_fast_1.8v_pu   GP io,fast slew,pu,1.8V
pio_fast_2.5v_pu   GP io,fast slew,pu,2.5V
pio_fast_3.3v_pu   GP io,fast slew,pu,3.3V
analog_1.8v   adc input 1.8v
analog_2.5v   adc input 2.5v
analog_3.3v   adc input 3.3v
[Model Selector]   pio1_4
pio_1.8v   GP io,1.8V
pio_2.5v   GP io,2.5V
pio_3.3v   GP io,3.3V
pio_1.8v_pd   GP io,pd,1.8V
pio_2.5v_pd   GP io,pd,2.5V
pio_3.3v_pd   GP io,pd,3.3V
pio_1.8v_pu   GP io,pu,1.8V | Pwrup Default
pio_2.5v_pu   GP io,pu,2.5V | Pwrup Default
pio_3.3v_pu   GP io,pu,3.3V | Pwrup Default
pio_fast_1.8v   GP io,fast slew,1.8V
pio_fast_2.5v   GP io,fast slew,2.5V
pio_fast_3.3v   GP io,fast slew,3.3V
pio_fast_1.8v_pd   GP io,fast slew,pd,1.8V
pio_fast_2.5v_pd   GP io,fast slew,pd,2.5V
pio_fast_3.3v_pd   GP io,fast slew,pd,3.3V
pio_fast_1.8v_pu   GP io,fast slew,pu,1.8V
pio_fast_2.5v_pu   GP io,fast slew,pu,2.5V
pio_fast_3.3v_pu   GP io,fast slew,pu,3.3V
analog_1.8v   adc input 1.8v
analog_2.5v   adc input 2.5v
analog_3.3v   adc input 3.3v
[Model Selector]   pio1_5
pio_1.8v   GP io,1.8V
pio_2.5v   GP io,2.5V
pio_3.3v   GP io,3.3V
pio_1.8v_pd   GP io,pd,1.8V
pio_2.5v_pd   GP io,pd,2.5V
pio_3.3v_pd   GP io,pd,3.3V
pio_1.8v_pu   GP io,pu,1.8V | Pwrup Default
pio_2.5v_pu   GP io,pu,2.5V | Pwrup Default
pio_3.3v_pu   GP io,pu,3.3V | Pwrup Default
pio_fast_1.8v   GP io,fast slew,1.8V
pio_fast_2.5v   GP io,fast slew,2.5V
pio_fast_3.3v   GP io,fast slew,3.3V
pio_fast_1.8v_pd   GP io,fast slew,pd,1.8V
pio_fast_2.5v_pd   GP io,fast slew,pd,2.5V
pio_fast_3.3v_pd   GP io,fast slew,pd,3.3V
pio_fast_1.8v_pu   GP io,fast slew,pu,1.8V
pio_fast_2.5v_pu   GP io,fast slew,pu,2.5V
pio_fast_3.3v_pu   GP io,fast slew,pu,3.3V
analog_1.8v   adc input 1.8v
analog_2.5v   adc input 2.5v
analog_3.3v   adc input 3.3v
[Model Selector]   pio1_6
pio_1.8v   GP io,1.8V
pio_2.5v   GP io,2.5V
pio_3.3v   GP io,3.3V
pio_1.8v_pd   GP io,pd,1.8V
pio_2.5v_pd   GP io,pd,2.5V
pio_3.3v_pd   GP io,pd,3.3V
pio_1.8v_pu   GP io,pu,1.8V | Pwrup Default
pio_2.5v_pu   GP io,pu,2.5V | Pwrup Default
pio_3.3v_pu   GP io,pu,3.3V | Pwrup Default
pio_fast_1.8v   GP io,fast slew,1.8V
pio_fast_2.5v   GP io,fast slew,2.5V
pio_fast_3.3v   GP io,fast slew,3.3V
pio_fast_1.8v_pd   GP io,fast slew,pd,1.8V
pio_fast_2.5v_pd   GP io,fast slew,pd,2.5V
pio_fast_3.3v_pd   GP io,fast slew,pd,3.3V
pio_fast_1.8v_pu   GP io,fast slew,pu,1.8V
pio_fast_2.5v_pu   GP io,fast slew,pu,2.5V
pio_fast_3.3v_pu   GP io,fast slew,pu,3.3V
analog_1.8v   adc input 1.8v
analog_2.5v   adc input 2.5v
analog_3.3v   adc input 3.3v
[Model Selector]   pio1_7
pio_1.8v   GP io,1.8V
pio_2.5v   GP io,2.5V
pio_3.3v   GP io,3.3V
pio_1.8v_pd   GP io,pd,1.8V
pio_2.5v_pd   GP io,pd,2.5V
pio_3.3v_pd   GP io,pd,3.3V
pio_1.8v_pu   GP io,pu,1.8V | Pwrup Default
pio_2.5v_pu   GP io,pu,2.5V | Pwrup Default
pio_3.3v_pu   GP io,pu,3.3V | Pwrup Default
pio_fast_1.8v   GP io,fast slew,1.8V
pio_fast_2.5v   GP io,fast slew,2.5V
pio_fast_3.3v   GP io,fast slew,3.3V
pio_fast_1.8v_pd   GP io,fast slew,pd,1.8V
pio_fast_2.5v_pd   GP io,fast slew,pd,2.5V
pio_fast_3.3v_pd   GP io,fast slew,pd,3.3V
pio_fast_1.8v_pu   GP io,fast slew,pu,1.8V
pio_fast_2.5v_pu   GP io,fast slew,pu,2.5V
pio_fast_3.3v_pu   GP io,fast slew,pu,3.3V
analog_1.8v   adc input 1.8v
analog_2.5v   adc input 2.5v
analog_3.3v   adc input 3.3v
[Model Selector]   pio1_8
pio_1.8v   GP io,1.8V
pio_2.5v   GP io,2.5V
pio_3.3v   GP io,3.3V
pio_1.8v_pd   GP io,pd,1.8V
pio_2.5v_pd   GP io,pd,2.5V
pio_3.3v_pd   GP io,pd,3.3V
pio_1.8v_pu   GP io,pu,1.8V | Pwrup Default
pio_2.5v_pu   GP io,pu,2.5V | Pwrup Default
pio_3.3v_pu   GP io,pu,3.3V | Pwrup Default
pio_fast_1.8v   GP io,fast slew,1.8V
pio_fast_2.5v   GP io,fast slew,2.5V
pio_fast_3.3v   GP io,fast slew,3.3V
pio_fast_1.8v_pd   GP io,fast slew,pd,1.8V
pio_fast_2.5v_pd   GP io,fast slew,pd,2.5V
pio_fast_3.3v_pd   GP io,fast slew,pd,3.3V
pio_fast_1.8v_pu   GP io,fast slew,pu,1.8V
pio_fast_2.5v_pu   GP io,fast slew,pu,2.5V
pio_fast_3.3v_pu   GP io,fast slew,pu,3.3V
analog_1.8v   adc input 1.8v
analog_2.5v   adc input 2.5v
analog_3.3v   adc input 3.3v
|**Special function pins
[Model Selector]   analog_io
analog_1.8v   analog io,1.8V
analog_2.5v   analog io,2.5V
analog_3.3v   analog io,3.3V
[Model Selector]   reset
reset_1.8v   reset input,1.8V
reset_2.5v   reset input,2.5V
reset_3.3v   reset input,3.3V
[Model Selector]   rtcxin
rtcxin_1.8v   Real Time Clock in,analog pad,1.8V
rtcxin_2.5v   Real Time Clock in,analog pad,2.5V
rtcxin_3.3v   Real Time Clock in,analog pad,3.3V
[Model Selector]   rtcxout
rtcxout_1.8v   Real Time Clock out,analog pad,1.8V
rtcxout_2.5v   Real Time Clock out,analog pad,2.5V
rtcxout_3.3v   Real Time Clock out,analog pad,3.3V
| Models and submodels in the file (36): reset_1.8v (Input), reset_2.5v (Input), reset_3.3v (Input), i2c_norm_hi_1.8v (I/O_open_drain), i2c_norm_lo_1.8v (I/O_open_drain), i2c_norm_hi_2.5v (I/O_open_drain), i2c_norm_lo_2.5v (I/O_open_drain), i2c_norm_hi_3.3v (I/O_open_drain), i2c_norm_lo_3.3v (I/O_open_drain), pio_1.8v (I/O), pio_1.8v_pd (I/O), pio_1.8v_pu (I/O), pio_2.5v (I/O), pio_2.5v_pd (I/O), pio_2.5v_pu (I/O), pio_3.3v (I/O), pio_3.3v_pd (I/O), pio_3.3v_pu (I/O), pio_fast_1.8v (I/O), pio_fast_1.8v_pd (I/O), pio_fast_1.8v_pu (I/O), pio_fast_2.5v (I/O), pio_fast_2.5v_pd (I/O), pio_fast_2.5v_pu (I/O), pio_fast_3.3v (I/O), pio_fast_3.3v_pd (I/O), pio_fast_3.3v_pu (I/O), rtcxout_1.8v (Open_drain), rtcxout_2.5v (Open_drain), rtcxout_3.3v (Open_drain), analog_1.8v (Terminator), analog_2.5v (Terminator), analog_3.3v (Terminator), rtcxin_1.8v (Terminator), rtcxin_2.5v (Terminator), rtcxin_3.3v (Terminator)
